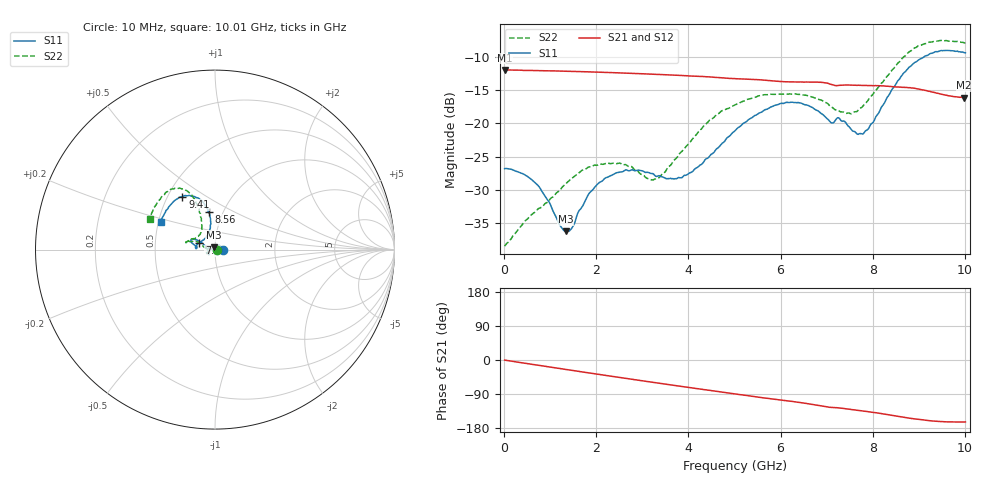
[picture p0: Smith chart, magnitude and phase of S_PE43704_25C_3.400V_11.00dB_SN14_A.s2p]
! Device ID: PE43704
! Dir: z:\PE43704\PE43704_Char_1_20130516\PE43704\AMB\3p400V\11p00dB
! Serial: 14
! Insertion: A
! Impedance: 50 ohm
! Temp: Amb
! VDD: 3.400V
! Attenuation Step: 11.00dB
! IDD: 1.140219e-01mA
#  Hz  S  RI  R  50
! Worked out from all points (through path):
!   401 points, 10 MHz to 10.01 GHz, reference 50 ohm
!   highest |S21| = -11.97 dB at 10 MHz (marker M1); lowest = -16.1 dB at 9.985 GHz (marker M2)
!   group delay of S21, straight-line fit = 47.1 ps
!   lowest |S11| = -36.2 dB at 1.335 GHz (marker M3), VSWR 1.03, Z = 49.2 + j1.34 ohm
!   |S11| at or under -10 dB: start of sweep to 9.113 GHz
!   |S22| runs from -38.4 to -7.5 dB; largest |S21 - S12| = 0.0019
!   S11 on the Smith chart (normalised r, x): 10 MHz: 1.10, +0.00; 7.46 GHz: 0.84, +0.06; 8.56 GHz: 0.86, +0.38; 9.41 GHz: 0.59, +0.40; 10.01 GHz: 0.51, +0.18
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1e7  0.0457 0.000342  0.2521 -0.00092  0.2522 -0.000824  0.0119 0.00042
7.1e8  0.027 0.022  0.2425 -0.0578  0.2424 -0.0577  -0.00321 0.0221
1.335e9  -0.00741 0.0136  0.2235 -0.1037  0.2236 -0.1036  -0.0329 0.0118
1.46e9  -0.0136 0.00877  0.2188 -0.1122  0.2188 -0.112  -0.0377 0.00693
1.685e9  -0.0234 8.41e-05  0.2092 -0.1271  0.2092 -0.127  -0.0442 -0.00235
2.01e9  -0.0323 -0.012  0.1935 -0.1466  0.1935 -0.1465  -0.0463 -0.0141
2.41e9  -0.0353 -0.023  0.1718 -0.1679  0.1719 -0.1679  -0.0454 -0.0212
3.16e9  -0.0331 -0.0264  0.1256 -0.1984  0.1258 -0.1982  -0.0365 -0.0108
3.36e9  -0.0338 -0.0223  0.1122 -0.2043  0.1124 -0.2042  -0.0388 -0.00409
4.035e9  -0.0426 0.00133  0.0661 -0.2171  0.0665 -0.2171  -0.0691 0.0209
4.46e9  -0.0536 0.0186  0.037 -0.2205  0.0374 -0.2205  -0.097 0.0427
5.01e9  -0.078 0.0409  0.00168 -0.2169  0.00181 -0.217  -0.1301 0.045
5.96e9  -0.1265 0.0588  -0.0535 -0.1996  -0.0529 -0.1997  -0.1595 0.0445
6.685e9  -0.1272 0.0353  -0.0926 -0.1822  -0.0927 -0.1818  -0.1505 0.0477
7.46e9  -0.0882 0.0377  -0.1231 -0.1502  -0.123 -0.1504  -0.0899 0.079
7.835e9  -0.0473 0.0735  -0.1374 -0.1351  -0.1374 -0.1354  -0.074 0.121
8.36e9  -0.0246 0.1634  -0.1552 -0.1087  -0.1546 -0.1093  -0.0878 0.2194
8.56e9  -0.035 0.2091  -0.1613 -0.096  -0.1604 -0.0966  -0.1075 0.2664
8.935e9  -0.0809 0.2775  -0.1667 -0.075  -0.1663 -0.0733  -0.1662 0.3321
9.41e9  -0.1821 0.2942  -0.1601 -0.0523  -0.1602 -0.0518  -0.2572 0.3267
9.985e9  -0.2979 0.1632  -0.15 -0.044  -0.1503 -0.0442  -0.3596 0.1791
1.001e10  -0.3027 0.1531  -0.1502 -0.0447  -0.151 -0.0451  -0.3633 0.1713
